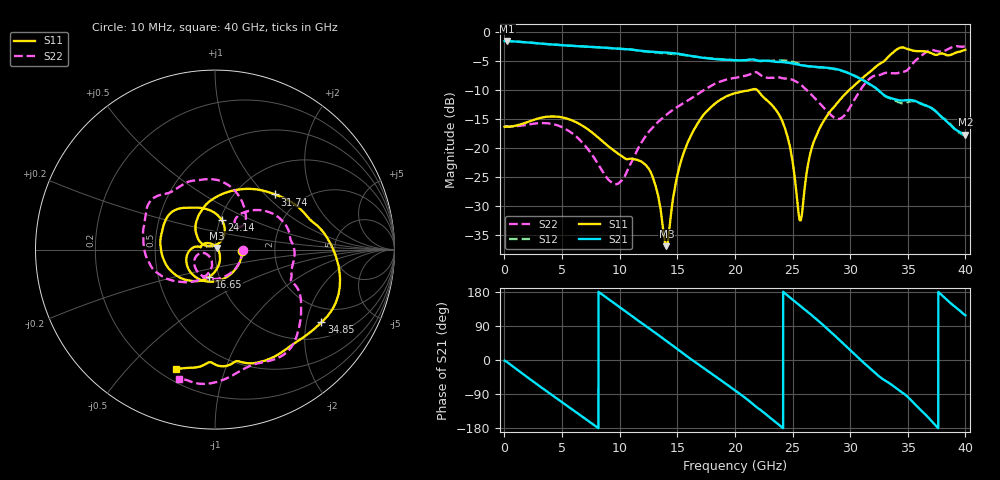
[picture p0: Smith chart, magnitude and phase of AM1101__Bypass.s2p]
!Agilent Technologies,E8364B,MY43040894,A.07.50.67
!Agilent E8364B: A.07.50.67
!Date: Tuesday, June 02, 2020 10:49:10
!Correction: S11(Full 2 Port(1,2))
!S21(Full 2 Port(1,2))
!S12(Full 2 Port(1,2))
!S22(Full 2 Port(1,2))
!S2P File: Measurements: S11, S21, S12, S22:
# Hz S  dB  R 50
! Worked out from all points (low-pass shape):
!   6401 points, 10 MHz to 40 GHz, reference 50 ohm
!   highest |S21| = -1.58 dB at 222.4 MHz (marker M1); lowest = -17.7 dB at 40 GHz (marker M2)
!   |S21| within 3 dB of the highest: start of sweep to 17.73 GHz
!   lowest |S11| = -36.8 dB at 14.04 GHz (marker M3), VSWR 1.03, Z = 51.2 + j0.874 ohm
!   |S11| at or under -10 dB: start of sweep to 21.34 GHz; 21.93 GHz to 29.93 GHz (8.004 GHz wide, 30.9 % of centre)
!   |S22| runs from -26.2 to -2.5 dB; largest |S21 - S12| = 0.024
!   S11 on the Smith chart (normalised r, x): 10 MHz: 1.36, -0.02; 16.65 GHz: 0.89, -0.28; 24.14 GHz: 1.02, +0.34; 31.74 GHz: 1.48, +1.14; 34.85 GHz: 1.47, -2.46; 40 GHz: 0.27, -0.69
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1e7  -16.34 -2.9  -1.60 -1.8  -1.49 -1.8  -16.20 -1.4
2.224469e8  -16.27 -9.3  -1.58 -5.4  -1.58 -5.4  -16.23 -8.8
3.446641e9  -14.66 -109.0  -2.08 -77.8  -2.07 -77.8  -15.68 -103.2
6.677083e9  -16.03 -169.4  -2.51 -147.9  -2.50 -147.9  -18.88 -159.7
9.751314e9  -20.79 169.3  -2.88 144.8  -2.87 144.6  -26.16 -132.1
1.145089e10  -21.98 167.0  -3.18 107.2  -3.20 106.6  -20.60 -100.4
1.334417e10  -28.27 122.7  -3.51 66.1  -3.62 65.9  -15.46 -112.7
1.404399e10  -36.84 36.4  -3.57 50.6  -3.71 50.7  -14.28 -118.6
1.516871e10  -23.31 -66.9  -3.80 24.8  -3.90 25.5  -12.71 -128.6
1.664959e10  -16.12 -102.3  -4.31 -7.9  -4.30 -7.1  -10.89 -142.2
2.0005e10  -10.55 -174.3  -4.87 -80.3  -4.88 -80.1  -7.91 173.0
2.157961e10  -9.88 149.1  -4.76 -116.8  -4.81 -116.3  -7.05 148.9
2.413522e10  -15.46 77.0  -5.20 -178.7  -4.91 -178.2  -8.00 104.5
2.484754e10  -20.47 57.0  -5.39 162.9  -5.08 162.5  -8.15 90.9
2.565359e10  -32.40 104.0  -5.70 142.8  -5.55 141.2  -8.98 74.1
2.667208e10  -19.93 150.7  -5.95 118.0  -6.00 117.0  -10.87 55.1
2.908398e10  -11.74 100.5  -6.55 52.3  -6.62 52.2  -14.94 50.4
3.173957e10  -6.85 42.6  -9.06 -22.3  -9.07 -23.0  -7.98 26.3
3.333917e10  -4.24 8.7  -11.28 -60.0  -11.33 -60.6  -7.09 -7.5
3.485129e10  -2.88 -34.3  -11.76 -93.5  -12.17 -92.0  -6.74 -22.5
3.668833e10  -3.44 -68.9  -12.75 -148.7  -12.75 -147.4  -3.36 -49.6
4e10  -3.10 -108.0  -17.65 117.9  -17.84 118.9  -2.50 -105.6
